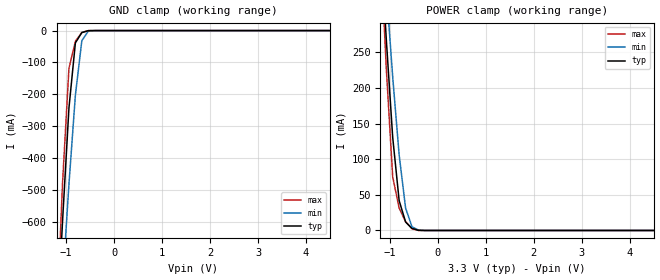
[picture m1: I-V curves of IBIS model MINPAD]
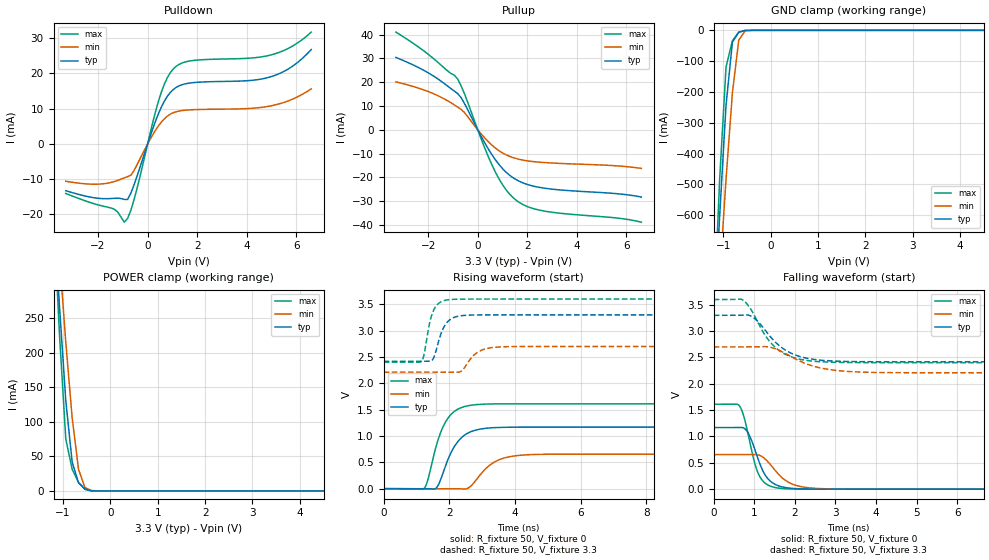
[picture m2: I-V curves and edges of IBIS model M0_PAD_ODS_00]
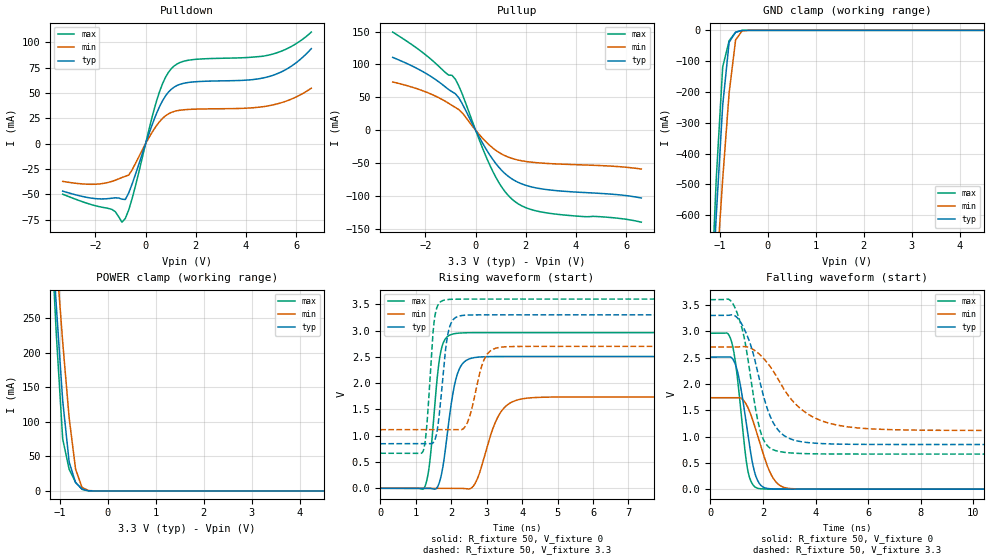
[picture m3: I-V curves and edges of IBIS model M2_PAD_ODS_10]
| Created by SiliconSmart  O-2018.09-SP2-3
[IBIS Ver]   4.0
[File Name]   as34b32bc_3p3_rev1p4.ibs
[File Rev]   1.4
[Date]   Thursday Mar 21 2024
|[Source]   Avalanche Team
|[Notes]   Generated IBIS models from Silicon Smart
|[Rev 1.0]  Initial Release based on extracted netlist
|   Characterization
|[Rev 1.1]  Recharacterization with Hspice, run in high accuracy mode
|[Rev 1.2]  Recharacterization with Hspice, parameters aligned with
|   datasheet
|[Rev 1.3]  Recharacterization with Hspice, run with updated VIH/VIL
|   in parallel with datasheet rev X.7
|[Rev 1.4]  Update the pin to the package pinout assignment
|[Disclaimer]   THE MODEL LIBRARIES ARE PROVIDED AS IS.
|[Copyright]   Copyright 2019, Avalanche Technology., All Rights Reserved
[Component]   AS304GB32_BGA
[Manufacturer] Avalanche Technology
| CONTENT :
| This file contains IBIS MODEL for PSRAM device
| AS304GB32
| USAGE :
| The models are derived for the 2.7V to 3.6V I/O Operation.
| Temperatures for model generation: typ: 25, max: -40, min: 125
| Voltages : typ: 3.3V, min: 2.7V, max: 3.6V
| PACKAGES SUPPORTED :
| 142-ball FBGA (15mm x 17mm)
| VERIFICATION
| Errors  : 0
| Warnings: 11
| All warnings due to non-monotonic data:
[Package]
R_pkg 0   0   0
L_pkg 0   0   0
C_pkg 0   0   0
[Pin]   signal_name   model_name   R_pin   L_pin   C_pin
P8   E#   MINPAD   0.254	7.307E-9	1.178E-12
P7   G#   MINPAD   0.243	7.052E-9	1.094E-12
J2   CR#   MINPAD   0.547	10.386E-9	1.789E-12
K3   PG#   MINPAD   0.451	10.329E-9	1.676E-12
M8   W#   MINPAD   0.377	9.020E-9	1.417E-12
M2   ADDR_26   MINPAD   0.425	9.037E-9	1.604E-12
L4   ADDR_25   MINPAD   0.419	9.644E-9	1.527E-12
K13   ADDR_24   MINPAD   0.495	9.978E-9	1.745E-12
M3   ADDR_23   MINPAD   0.371	9.313E-9	1.466E-12
L3   ADDR_22   MINPAD   0.412	9.753E-9	1.540E-12
M7   ADDR_21   MINPAD   0.368	8.765E-9	1.384E-12
P12   ADDR_20   MINPAD   0.287	8.287E-9	1.639E-12
L12   ADDR_19   MINPAD   0.424	10.320E-9	1.620E-12
N11   ADDR_18   MINPAD   0.338	8.691E-9	1.470E-12
N6   ADDR_17   MINPAD   0.309	8.196E-9	1.279E-12
P6   ADDR_16   MINPAD   0.256	7.462E-9	1.204E-12
L13   ADDR_15   MINPAD   0.463	10.719E-9	1.740E-12
M13   ADDR_14   MINPAD   0.421	10.290E-9	1.689E-12
P10   ADDR_13   MINPAD   0.262	7.671E-9	1.349E-12
N10   ADDR_12   MINPAD   0.340	8.540E-9	1.360E-12
M12   ADDR_11   MINPAD   0.402	9.876E-9	1.604E-12
N13   ADDR_10   MINPAD   0.399	9.819E-9	1.696E-12
L11   ADDR_9   MINPAD   0.443	9.732E-9	1.569E-12
M11   ADDR_8   MINPAD   0.436	9.682E-9	1.671E-12
P5   ADDR_7   MINPAD   0.253	7.464E-9	1.277E-12
P3   ADDR_6   MINPAD   0.279	8.031E-9	1.557E-12
N5   ADDR_5   MINPAD   0.313	8.320E-9	1.359E-12
N4   ADDR_4   MINPAD   0.329	8.138E-9	1.428E-12
M4   ADDR_3   MINPAD   0.379	8.543E-9	1.406E-12
N2   ADDR_2   MINPAD   0.378	9.572E-9	1.637E-12
N9   ADDR_1   MINPAD   0.315	8.416E-9	1.305E-12
M9   ADDR_0   MINPAD   0.403	9.225E-9	1.473E-12
E2   DQ_31   MIOPAD   0.365	8.798E-9	1.454E-12
F2   DQ_30   MIOPAD   0.418	9.057E-9	1.576E-12
D2   DQ_29   MIOPAD   0.358	8.697E-9	1.520E-12
E3   DQ_28   MIOPAD   0.348	8.812E-9	1.441E-12
E12   DQ_27   MIOPAD   0.327	8.506E-9	1.443E-12
D10   DQ_26   MIOPAD   0.309	7.715E-9	1.264E-12
C9   DQ_25   MIOPAD   0.279	7.395E-9	1.219E-12
C7   DQ_24   MIOPAD   0.252	6.802E-9	1.108E-12
G4   DQ_23   MIOPAD   0.455	10.071E-9	1.775E-12
G3   DQ_22   MIOPAD   0.457	10.100E-9	1.750E-12
F13   DQ_21   MIOPAD   0.377	9.387E-9	1.566E-12
D13   DQ_20   MIOPAD   0.295	8.231E-9	1.460E-12
C10   DQ_19   MIOPAD   0.293	7.553E-9	1.298E-12
E8   DQ_18   MIOPAD   0.393	8.323E-9	1.436E-12
F6   DQ_17   MIOPAD   0.425	8.913E-9	1.517E-12
E5   DQ_16   MIOPAD   0.379	8.982E-9	1.460E-12
E13   DQ_15   MIOPAD   0.363	8.555E-9	1.474E-12
G11   DQ_14   MIOPAD   0.475	9.536E-9	1.630E-12
E10   DQ_13   MIOPAD   0.404	8.563E-9	1.453E-12
F9   DQ_12   MIOPAD   0.409	9.347E-9	1.513E-12
C8   DQ_11   MIOPAD   0.257	6.782E-9	1.111E-12
C6   DQ_10   MIOPAD   0.238	7.000E-9	1.114E-12
D6   DQ_9   MIOPAD   0.292	7.776E-9	1.248E-12
D4   DQ_8   MIOPAD   0.305	7.782E-9	1.343E-12
G12   DQ_7   MIOPAD   0.502	10.055E-9	1.687E-12
C12   DQ_6   MIOPAD   0.275	7.857E-9	1.346E-12
D11   DQ_5   MIOPAD   0.286	7.835E-9	1.360E-12
D9   DQ_4   MIOPAD   0.306	8.035E-9	1.299E-12
E7   DQ_3   MIOPAD   0.384	8.178E-9	1.375E-12
C5   DQ_2   MIOPAD   0.231	6.786E-9	1.150E-12
D5   DQ_1   MIOPAD   0.307	7.698E-9	1.346E-12
C3   DQ_0   MIOPAD   0.267	7.420E-9	1.241E-12
G13   INT#   MIOPAD   0.480	10.704E-9	1.759E-12
F10   VSSIO   GND   NA   NA   NA
L10   VSSIO   GND   NA   NA   NA
E9   VSSIO   GND   NA   NA   NA
L9   VSSIO   GND   NA   NA   NA
F8   VSSIO   GND   NA   NA   NA
L8   VSSIO   GND   NA   NA   NA
F7   VSSIO   GND   NA   NA   NA
L7   VSSIO   GND   NA   NA   NA
E6   VSSIO   GND   NA   NA   NA
L6   VSSIO   GND   NA   NA   NA
G5   VSSIO   GND   NA   NA   NA
A14   VSS   GND   NA   NA   NA
B14   VSS   GND   NA   NA   NA
C14   VSS   GND   NA   NA   NA
H13   VSS   GND   NA   NA   NA
R14   VSS   GND   NA   NA   NA
T14   VSS   GND   NA   NA   NA
A13   VSS   GND   NA   NA   NA
T13   VSS   GND   NA   NA   NA
A12   VSS   GND   NA   NA   NA
G10   VSS   GND   NA   NA   NA
H10   VSS   GND   NA   NA   NA
J10   VSS   GND   NA   NA   NA
K10   VSS   GND   NA   NA   NA
F5   VSS   GND   NA   NA   NA
L5   VSS   GND   NA   NA   NA
A2   VSS   GND   NA   NA   NA
T2   VSS   GND   NA   NA   NA
A1   VSS   GND   NA   NA   NA
B1   VSS   GND   NA   NA   NA
R1   VSS   GND   NA   NA   NA
T1   VSS   GND   NA   NA   NA
F12   VCCIO   POWER   NA   NA   NA
J12   VCCIO   POWER   NA   NA   NA
E11   VCCIO   POWER   NA   NA   NA
M10   VCCIO   POWER   NA   NA   NA
D8   VCCIO   POWER   NA   NA   NA
N8   VCCIO   POWER   NA   NA   NA
D7   VCCIO   POWER   NA   NA   NA
N7   VCCIO   POWER   NA   NA   NA
M5   VCCIO   POWER   NA   NA   NA
E4   VCCIO   POWER   NA   NA   NA
F3   VCCIO   POWER   NA   NA   NA
J3   VCCIO   POWER   NA   NA   NA
C13   VCC   POWER   NA   NA   NA
P13   VCC   POWER   NA   NA   NA
D12   VCC   POWER   NA   NA   NA
N12   VCC   POWER   NA   NA   NA
C11   VCC   POWER   NA   NA   NA
F11   VCC   POWER   NA   NA   NA
H11   VCC   POWER   NA   NA   NA
J11   VCC   POWER   NA   NA   NA
K11   VCC   POWER   NA   NA   NA
P11   VCC   POWER   NA   NA   NA
C4   VCC   POWER   NA   NA   NA
F4   VCC   POWER   NA   NA   NA
H4   VCC   POWER   NA   NA   NA
J4   VCC   POWER   NA   NA   NA
K4   VCC   POWER   NA   NA   NA
P4   VCC   POWER   NA   NA   NA
D3   VCC   POWER   NA   NA   NA
N3   VCC   POWER   NA   NA   NA
C2   VCC   POWER   NA   NA   NA
P2   VCC   POWER   NA   NA   NA
| IOPAD
[Model Selector] MIOPAD
| Model Description
M0_PAD_ODS_00   ODS_00
M1_PAD_ODS_01   ODS_01
M2_PAD_ODS_10   ODS_10
M3_PAD_ODS_11   ODS_11
| Models and submodels in the file (5): MINPAD (Input), M0_PAD_ODS_00 (I/O), M2_PAD_ODS_10 (I/O), M1_PAD_ODS_01 (I/O), M3_PAD_ODS_11 (I/O)
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| INPAD
[Model] MINPAD
Model_type Input
Enable   Active-High
Vinl  =  0.8
Vinh  =  2.2
| Capacitance  typ   min   max
C_comp   6.059285e-12   5.673711e-12   6.587901e-12
| Variables   typ   min   max
[GND Clamp Reference]   0   0   0
[POWER Clamp Reference]   3.3   2.7   3.6
[Pulldown Reference]   0   0   0
[Pullup Reference]   3.3   2.7   3.6
[Temperature Range]   25   125   -40
[Voltage Range]   3.3   2.7   3.6
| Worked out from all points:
|   GND clamp passes 1 mA (typ) near -0.55 V on its own axis
|   POWER clamp passes 1 mA (typ) near -0.44 V on its own axis
[GND Clamp]
| Voltage   I(typ)   I(min)   I(max)
-3.3V     -7.845A    -6.789A    -9.429A
-1.21V    -1.003A    -1.135A    -969.9mA
-1.076V   -602.2mA   -800.5mA   -482.6mA
-941.4mV  -243.3mA   -483.1mA   -119mA
-806.9mV  -38.58mA   -202.8mA   -33.74mA
-672.4mV  -6.342mA   -31.46mA   -5.828mA
-537.9mV  -287uA     -2.017mA   -74.91uA
-403.4mV  -2.376uA   -74.29uA   -148.9nA
6.6V      0A         0A         0A
[POWER Clamp]
| Voltage   I(typ)   I(min)   I(max)
-3.3V     3.089A     2.693A     3.722A
-1.21V    423.7mA    470.3mA    418.3mA
-1.076V   269.4mA    340.2mA    228.7mA
-941.4mV  130.8mA    215.7mA    75.29mA
-806.9mV  41.91mA    106.1mA    31.39mA
-672.4mV  11.9mA     31.42mA    12.43mA
-537.9mV  2.843mA    4.992mA    2.292mA
-403.4mV  242.8uA    643.4uA    36.75uA
-269mV    569.5nA    24.47uA    93.03nA
6.6V      0A         0A         0A
[Model] M0_PAD_ODS_00
Model_type I/O
Enable   Active-High
Vinl  =  0.8
Vinh  =  2.2
Vmeas =  1.65
Cref  =  30e-12
| Capacitance  typ   min   max
C_comp   6.058162e-12   5.681079e-12   6.591827e-12
| Variables   typ   min   max
[GND Clamp Reference]   0   0   0
[POWER Clamp Reference]   3.3   2.7   3.6
[Pulldown Reference]   0   0   0
[Pullup Reference]   3.3   2.7   3.6
[Temperature Range]   25   125   -40
[Voltage Range]   3.3   2.7   3.6
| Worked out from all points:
|   slope of the pulldown table from 0 to 0.495 V, typ, clamps not added: 52.1 ohm
|   slope of the pullup table from 0 to 0.495 V, typ, clamps not added: 53.8 ohm
|   GND clamp passes 1 mA (typ) near -0.55 V on its own axis
|   POWER clamp passes 1 mA (typ) near -0.44 V on its own axis
|   falling waveform, R_fixture 50, V_fixture 0: 20-80 % time 372ps typ, 511ps min, 310ps max; typ from 1.17 V to 0 V
|   falling waveform, R_fixture 50, V_fixture 3.3: 20-80 % time 714ps typ, 889ps min, 639ps max; typ from 3.3 V to 2.42 V
|   rising waveform, R_fixture 50, V_fixture 0: 20-80 % time 546ps typ, 658ps min, 498ps max; typ from 0 V to 1.17 V
|   rising waveform, R_fixture 50, V_fixture 3.3: 20-80 % time 304ps typ, 421ps min, 242ps max; typ from 2.42 V to 3.3 V
[GND Clamp]
| Voltage   I(typ)   I(min)   I(max)
-3.3V     -7.845A    -6.789A    -9.429A
-1.21V    -1.003A    -1.135A    -970mA
-1.076V   -602.2mA   -800.5mA   -482.6mA
-941.4mV  -243.3mA   -483.1mA   -119mA
-806.9mV  -38.59mA   -202.8mA   -33.75mA
-672.4mV  -6.344mA   -31.46mA   -5.83mA
-537.9mV  -287.2uA   -2.017mA   -75.02uA
-403.4mV  -2.377uA   -74.3uA    -149.1nA
6.6V      0A         0A         0A
[POWER Clamp]
| Voltage   I(typ)   I(min)   I(max)
-3.3V     3.089A     2.693A     3.722A
-1.21V    423.7mA    470.3mA    418.3mA
-1.076V   269.4mA    340.2mA    228.7mA
-941.4mV  130.8mA    215.7mA    75.29mA
-806.9mV  41.91mA    106.1mA    31.39mA
-672.4mV  11.9mA     31.42mA    12.43mA
-537.9mV  2.843mA    4.992mA    2.292mA
-403.4mV  242.8uA    643.4uA    36.75uA
-269mV    569.5nA    24.47uA    93.03nA
6.6V      0A         0A         0A
[Pulldown]
| Voltage   I(typ)   I(min)   I(max)
-3.3V     -13.26mA   -10.58mA   -14.05mA
-1.345V   -15.42mA   -10.67mA   -18.51mA
-941.4mV  -15.74mA   -9.611mA   -22.19mA
-806.9mV  -15.73mA   -9.263mA   -21.14mA
-537.9mV  -11.42mA   -7.417mA   -15.59mA
455.2mV   8.881mA    5.308mA    12.55mA
682.8mV   12.23mA    7.205mA    17.1mA
1.024V    15.38mA    8.837mA    21.2mA
1.821V    17.39mA    9.724mA    23.68mA
4.914V    18.96mA    10.73mA    25.16mA
5.783V    21.77mA    12.53mA    27.53mA
6.6V      26.8mA     15.66mA    31.75mA
[Pullup]
| Voltage   I(typ)   I(min)   I(max)
-3.3V     30.44mA    20.14mA    41.1mA
-1.883V   23.26mA    15.61mA    30.81mA
-806.9mV  15.23mA    9.539mA    21.27mA
-537.9mV  11.14mA    7.294mA    15.26mA
227.6mV   -4.448mA   -2.796mA   -6.209mA
682.8mV   -12.17mA   -7.42mA    -17.15mA
1.138V    -17.78mA   -10.49mA   -25.16mA
1.593V    -21.21mA   -12.21mA   -29.96mA
2.048V    -23.14mA   -13.13mA   -32.47mA
2.731V    -24.61mA   -13.8mA    -34.27mA
5.659V    -26.92mA   -15.2mA    -37.16mA
6.6V      -28.29mA   -16.23mA   -38.86mA
[Ramp]
dV/dt_r   0.701574/0.545719n  0.393696/0.658178n  0.967082/0.498225n
dV/dt_f   0.529394/0.71378n  0.294233/0.889277n  0.719381/0.63933n
R_load = 50
[Falling Waveform]
R_fixture = 50
V_fixture = 0
V_fixture_min = 0
V_fixture_max = 0
| Time   V(typ)   V(min)   V(max)
0s        1.169V     656.2mV    1.612V
634.8ps   1.17V      656.7mV    1.579V
865.5ps   1.041V     656.9mV    976.9mV
1.014ns   748.6mV    657.3mV    480.2mV
1.125ns   502.1mV    642.6mV    251.3mV
1.341ns   192.7mV    514.7mV    76.33mV
1.655ns   49.28mV    237.1mV    14.65mV
2.145ns   6.355mV    48.76mV    1.268mV
2.985ns   527.1uV    3.26mV     186.7uV
21.88ns   35.25nV    448.9nV    -1.236uV
[Falling Waveform]
R_fixture = 50
V_fixture = 3.3
V_fixture_min = 2.7
V_fixture_max = 3.6
| Time   V(typ)   V(min)   V(max)
0s        3.3V       2.7V       3.6V
723.6ps   3.304V     2.701V     3.588V
995.4ps   3.247V     2.701V     3.305V
1.255ns   3.03V      2.706V     2.934V
1.554ns   2.765V     2.655V     2.666V
1.968ns   2.559V     2.49V      2.498V
2.562ns   2.454V     2.313V     2.422V
3.327ns   2.424V     2.234V     2.404V
4.529ns   2.418V     2.212V     2.401V
21.88ns   2.418V     2.21V      2.401V
[Rising Waveform]
R_fixture = 50
V_fixture = 0
V_fixture_min = 0
V_fixture_max = 0
| Time   V(typ)   V(min)   V(max)
0s        43.53nV    350.8nV    65.75nV
1.224ns   -607.7uV   -367.6uV   -154.8uV
1.341ns   -665.8uV   -402.7uV   154.3mV
1.599ns   11.59mV    -480.3uV   804.9mV
1.893ns   447.6mV    -568.8uV   1.276V
2.331ns   945.5mV    -2.521mV   1.531V
2.813ns   1.113V     161.1mV    1.596V
3.412ns   1.16V      518.7mV    1.61V
4.362ns   1.169V     643.3mV    1.611V
21.88ns   1.169V     656.2mV    1.612V
[Rising Waveform]
R_fixture = 50
V_fixture = 3.3
V_fixture_min = 2.7
V_fixture_max = 3.6
| Time   V(typ)   V(min)   V(max)
0s        2.418V     2.21V      2.401V
1.143ns   2.419V     2.21V      2.412V
1.221ns   2.419V     2.21V      2.521V
1.528ns   2.49V      2.21V      3.397V
1.77ns    2.983V     2.21V      3.555V
1.984ns   3.19V      2.211V     3.588V
2.353ns   3.283V     2.229V     3.599V
2.966ns   3.299V     2.625V     3.6V
3.626ns   3.3V       2.694V     3.6V
21.88ns   3.3V       2.7V       3.6V
[Model] M2_PAD_ODS_10
Model_type I/O
Enable   Active-High
Vinl  =  0.8
Vinh  =  2.2
Vmeas =  1.65
Cref  =  30e-12
| Capacitance  typ   min   max
C_comp   6.058162e-12   5.681079e-12   6.591827e-12
| Variables   typ   min   max
[GND Clamp Reference]   0   0   0
[POWER Clamp Reference]   3.3   2.7   3.6
[Pulldown Reference]   0   0   0
[Pullup Reference]   3.3   2.7   3.6
[Temperature Range]   25   125   -40
[Voltage Range]   3.3   2.7   3.6
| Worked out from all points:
|   slope of the pulldown table from 0 to 0.495 V, typ, clamps not added: 14.9 ohm
|   slope of the pullup table from 0 to 0.495 V, typ, clamps not added: 14.7 ohm
|   GND clamp passes 1 mA (typ) near -0.55 V on its own axis
|   POWER clamp passes 1 mA (typ) near -0.44 V on its own axis
|   falling waveform, R_fixture 50, V_fixture 0: 20-80 % time 471ps typ, 687ps min, 384ps max; typ from 2.51 V to 0 V
|   falling waveform, R_fixture 50, V_fixture 3.3: 20-80 % time 833ps typ, 1.5ns min, 599ps max; typ from 3.3 V to 0.848 V
|   rising waveform, R_fixture 50, V_fixture 0: 20-80 % time 319ps typ, 518ps min, 240ps max; typ from 0 V to 2.51 V
|   rising waveform, R_fixture 50, V_fixture 3.3: 20-80 % time 222ps typ, 342ps min, 175ps max; typ from 0.848 V to 3.3 V
[GND Clamp]
| Voltage   I(typ)   I(min)   I(max)
-3.3V     -7.845A    -6.789A    -9.429A
-1.21V    -1.003A    -1.135A    -970mA
-1.076V   -602.2mA   -800.5mA   -482.6mA
-941.4mV  -243.3mA   -483.1mA   -119mA
-806.9mV  -38.59mA   -202.8mA   -33.75mA
-672.4mV  -6.344mA   -31.46mA   -5.83mA
-537.9mV  -287.2uA   -2.017mA   -75.02uA
-403.4mV  -2.377uA   -74.3uA    -149.1nA
6.6V      0A         0A         0A
[POWER Clamp]
| Voltage   I(typ)   I(min)   I(max)
-3.3V     3.089A     2.693A     3.722A
-1.21V    423.7mA    470.3mA    418.3mA
-1.076V   269.4mA    340.2mA    228.7mA
-941.4mV  130.8mA    215.7mA    75.29mA
-806.9mV  41.91mA    106.1mA    31.39mA
-672.4mV  11.9mA     31.42mA    12.43mA
-537.9mV  2.843mA    4.992mA    2.292mA
-403.4mV  242.8uA    643.4uA    36.75uA
-269mV    569.5nA    24.47uA    93.03nA
6.6V      0A         0A         0A
[Pulldown]
| Voltage   I(typ)   I(min)   I(max)
-3.3V     -46.77mA   -37.16mA   -49.83mA
-1.345V   -53.76mA   -37.21mA   -64.77mA
-941.4mV  -54.71mA   -33.33mA   -77.43mA
-806.9mV  -55.02mA   -32.17mA   -73.73mA
-537.9mV  -39.9mA    -25.92mA   -54.28mA
455.2mV   31.02mA    18.55mA    43.7mA
682.8mV   42.73mA    25.18mA    59.65mA
1.024V    53.77mA    30.89mA    74.07mA
1.821V    60.81mA    33.99mA    82.81mA
4.914V    66.31mA    37.51mA    87.55mA
5.783V    76.16mA    43.8mA     95.68mA
6.6V      93.82mA    54.81mA    110.2mA
[Pullup]
| Voltage   I(typ)   I(min)   I(max)
-3.3V     110.8mA    73.4mA     149.4mA
-1.883V   84.27mA    56.72mA    111.4mA
-806.9mV  55.48mA    34.56mA    77.7mA
-537.9mV  40.72mA    26.67mA    55.72mA
227.6mV   -16.26mA   -10.22mA   -22.67mA
682.8mV   -44.48mA   -27.12mA   -62.65mA
1.138V    -65.01mA   -38.35mA   -91.97mA
1.593V    -77.56mA   -44.65mA   -109.6mA
2.162V    -85.85mA   -48.54mA   -120.3mA
2.845V    -90.61mA   -50.73mA   -126.1mA
5.534V    -97.91mA   -55.15mA   -133.7mA
6.6V      -103.4mA   -59.29mA   -140.2mA
[Ramp]
dV/dt_r   1.50494/0.319227n  1.04234/0.518069n  1.77705/0.239679n
dV/dt_f   1.47119/0.833179n  0.951014/1.49863n  1.76015/0.599415n
R_load = 50
[Falling Waveform]
R_fixture = 50
V_fixture = 0
V_fixture_min = 0
V_fixture_max = 0
| Time   V(typ)   V(min)   V(max)
0s        2.508V     1.737V     2.962V
796.3ps   2.502V     1.738V     2.824V
924.1ps   2.408V     1.738V     2.522V
1.078ns   2.143V     1.739V     1.909V
1.409ns   1.111V     1.573V     401.1mV
1.599ns   510.8mV    1.335V     101.1mV
1.777ns   188mV      1.052V     19.7mV
2.393ns   4.468mV    206.2mV    1.223mV
3.049ns   938.6uV    10.99mV    368.5uV
21.88ns   -1.372uV   189.6nV    1.903uV
[Falling Waveform]
R_fixture = 50
V_fixture = 3.3
V_fixture_min = 2.7
V_fixture_max = 3.6
| Time   V(typ)   V(min)   V(max)
0s        3.3V       2.7V       3.6V
707.6ps   3.302V     2.7V       3.605V
978.1ps   3.279V     2.701V     3.404V
1.327ns   3.005V     2.707V     2.784V
1.897ns   2.02V      2.549V     1.115V
2.114ns   1.612V     2.433V     859.9mV
2.481ns   1.19V      2.172V     732.4mV
3.5ns     898.6mV    1.501V     676.3mV
5.249ns   852.8mV    1.182V     667mV
21.88ns   848mV      1.115V     666.4mV
[Rising Waveform]
R_fixture = 50
V_fixture = 0
V_fixture_min = 0
V_fixture_max = 0
| Time   V(typ)   V(min)   V(max)
0s        19.19nV    176.5nV    26.52nV
1.25ns    -561.1uV   -384.8uV   19.65mV
1.404ns   -630uV     -432.1uV   544.7mV
1.686ns   153mV      -518.8uV   2.527V
2.052ns   1.817V     -631.6uV   2.936V
2.494ns   2.458V     -12.96mV   2.96V
2.74ns    2.494V     182.6mV    2.961V
3.377ns   2.507V     1.427V     2.961V
4.147ns   2.507V     1.715V     2.961V
21.88ns   2.508V     1.737V     2.962V
[Rising Waveform]
R_fixture = 50
V_fixture = 3.3
V_fixture_min = 2.7
V_fixture_max = 3.6
| Time   V(typ)   V(min)   V(max)
0s        848mV      1.115V     666.4mV
1.213ns   847.5mV    1.114V     714.9mV
1.309ns   847.4mV    1.114V     1.166V
1.522ns   896.3mV    1.114V     3.19V
1.804ns   2.395V     1.114V     3.581V
2.108ns   3.241V     1.114V     3.598V
2.467ns   3.296V     1.266V     3.6V
2.966ns   3.3V       2.498V     3.6V
3.426ns   3.3V       2.686V     3.6V
21.88ns   3.3V       2.7V       3.6V
